(* Logix 5000 AddOnInstructionDefinition export FRA7NWIE_ACDC_Drive_Profile; software revision 19.01 *)

ADD_ON_INSTRUCTION FRA7NWIE_ACDC_Drive_Profile   (* revision 1.0 *)
// Interface for AC/DC Drive Profile that uses Input Assembly Instance 71 and Output Assembly Instance 21.
VAR_IN_OUT
   I_Data : INT[2]; {required}   // Input data
   O_Data : INT[2]; {required}   // Output data
END_VAR
VAR_INPUT
   RunForward : BOOL; {required}   // Run forward
   RunReverse : BOOL; {required}   // Run reverse
   ResetFault : BOOL; {required}   // Reset fault
   NetControl : BOOL; {required}   // Control from network
   NetReference : BOOL; {required}   // Speed reference from network
   SpeedReference : INT; {access Read Only, required}   // Speed reference (RPM)
END_VAR
VAR_OUTPUT
   Faulted : BOOL; {access Read Only, visible}   // Faulted
   RunningForward : BOOL; {access Read Only, visible}   // Running forward
   RunningReverse : BOOL; {access Read Only, visible}   // Running reverse
   Ready : BOOL; {access Read Only, visible}   // Ready
END_VAR
VAR_INPUT
   ControlFromNet : BOOL; {visible}   // Controlled from network
   ReferenceFromNet : BOOL; {visible}   // Speed referenced from network
END_VAR
VAR_OUTPUT
   AtReference : BOOL; {access Read Only, visible}   // Up-to-speed
   DriveState : SINT; {access Read Only, visible}   // Drive state (0 = vendor specific, 1 = startup, 2 = not ready, 3 = ready, 4 = enabled, 5 = stopping, 6 = fault stop, 7 = faulted)
   SpeedActual : INT; {access Read Only, visible}   // Actual speed (RPM)
END_VAR
VAR
   temp : INT; {access None}
END_VAR

ROUTINE Logic   (* ladder *)
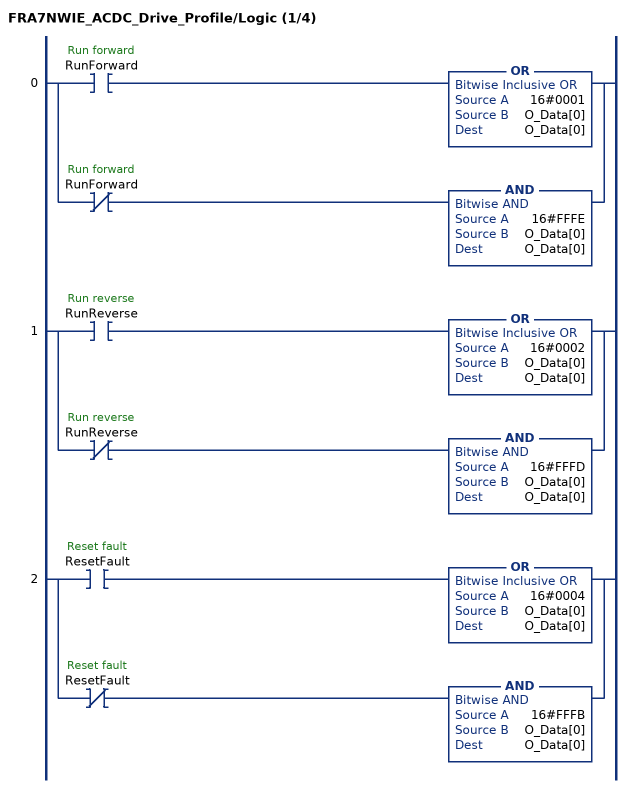
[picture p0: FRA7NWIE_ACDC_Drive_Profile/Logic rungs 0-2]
   0: [XIC(RunForward) OR(16#0001,O_Data[0],O_Data[0]) ,XIO(RunForward) AND(16#FFFE,O_Data[0],O_Data[0]) ];
   1: [XIC(RunReverse) OR(16#0002,O_Data[0],O_Data[0]) ,XIO(RunReverse) AND(16#FFFD,O_Data[0],O_Data[0]) ];
   2: [XIC(ResetFault) OR(16#0004,O_Data[0],O_Data[0]) ,XIO(ResetFault) AND(16#FFFB,O_Data[0],O_Data[0]) ];
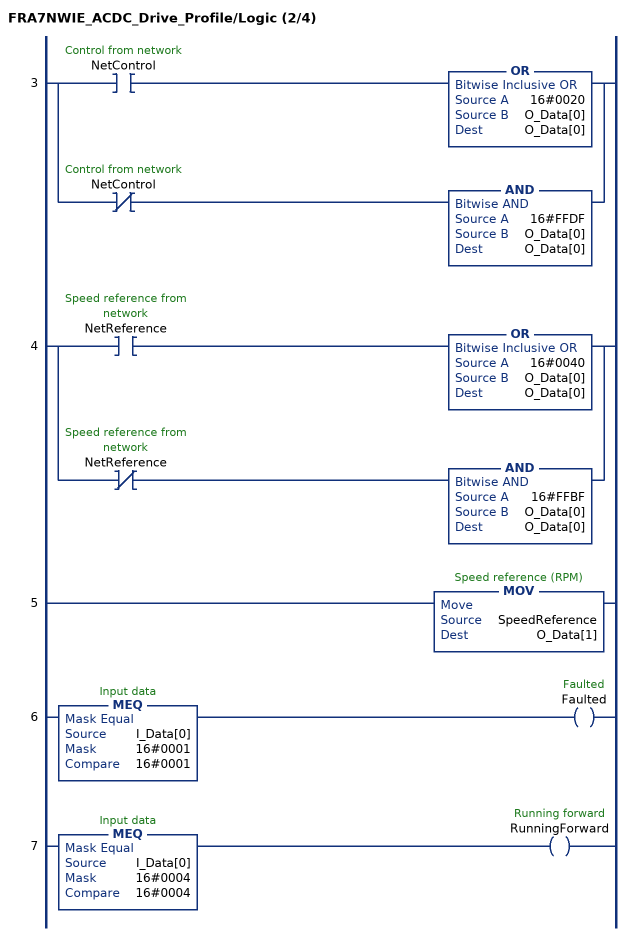
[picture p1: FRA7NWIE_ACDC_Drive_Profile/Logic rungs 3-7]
   3: [XIC(NetControl) OR(16#0020,O_Data[0],O_Data[0]) ,XIO(NetControl) AND(16#FFDF,O_Data[0],O_Data[0]) ];
   4: [XIC(NetReference) OR(16#0040,O_Data[0],O_Data[0]) ,XIO(NetReference) AND(16#FFBF,O_Data[0],O_Data[0]) ];
   5: MOV(SpeedReference,O_Data[1]);
   6: MEQ(I_Data[0],16#0001,16#0001)OTE(Faulted);
   7: MEQ(I_Data[0],16#0004,16#0004)OTE(RunningForward);
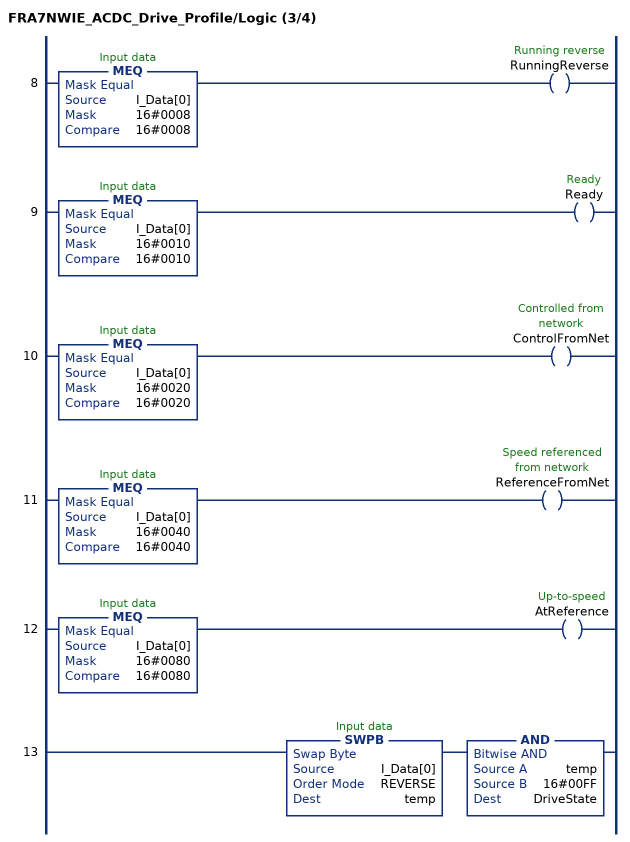
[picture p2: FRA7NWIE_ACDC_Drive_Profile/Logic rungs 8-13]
   8: MEQ(I_Data[0],16#0008,16#0008)OTE(RunningReverse);
   9: MEQ(I_Data[0],16#0010,16#0010)OTE(Ready);
   10: MEQ(I_Data[0],16#0020,16#0020)OTE(ControlFromNet);
   11: MEQ(I_Data[0],16#0040,16#0040)OTE(ReferenceFromNet);
   12: MEQ(I_Data[0],16#0080,16#0080)OTE(AtReference);
   13: SWPB(I_Data[0],REVERSE,temp)AND(temp,16#00FF,DriveState);
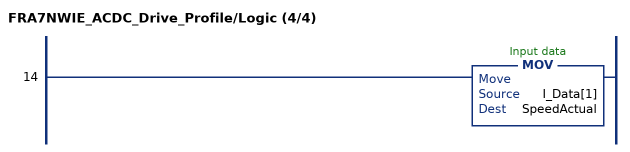
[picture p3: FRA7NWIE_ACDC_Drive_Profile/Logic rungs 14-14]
   14: MOV(I_Data[1],SpeedActual);
END_ROUTINE
END_ADD_ON_INSTRUCTION
